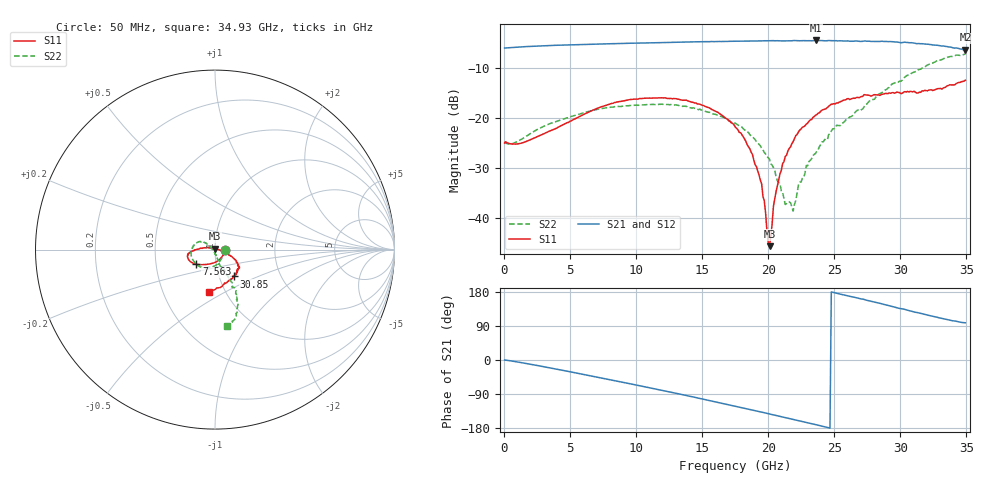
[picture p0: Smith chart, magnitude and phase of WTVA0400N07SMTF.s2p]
! 50 ohm 2-Port S-parameters measured by Modelithics Inc support@modelithics.com  Tampa, FL USA 813-866-6335 (February 2024)
! Smiths Interconnect,  4dB P/N: WTVA0400N07SMTF, Temperature: -25 C
! Board: 10 mil Rogers 4350B, Mounting Pad Dimensions: Length: 15 mils, Width: 25 mils, Gap: 40 mils.
# Hz S RI R 50
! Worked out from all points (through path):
!   352 points, 50 MHz to 34.93 GHz, reference 50 ohm
!   highest |S21| = -4.56 dB at 23.58 GHz (marker M1); lowest = -6.4 dB at 34.93 GHz (marker M2)
!   group delay of S21, straight-line fit = 21.3 ps
!   lowest |S11| = -45.6 dB at 20.1 GHz (marker M3), VSWR 1.01, Z = 50.1 + j0.521 ohm
!   |S11| at or under -10 dB: start of sweep to end of sweep
!   |S22| runs from -38.6 to -7.3 dB; largest |S21 - S12| = 0.0056
!   S11 on the Smith chart (normalised r, x): 50 MHz: 1.12, -0.01; 7.563 GHz: 0.80, -0.13; 30.85 GHz: 1.18, -0.36; 34.93 GHz: 0.84, -0.42
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5e7  0.0563 -0.00229  0.4972 -0.0006  0.4965 -0.000787  0.0576 -0.00224
5.8715e9  -0.0645 -0.0838  0.4309 -0.3249  0.4301 -0.3248  -0.0439 -0.1015
7.563e9  -0.1033 -0.081  0.3607 -0.411  0.3594 -0.4112  -0.0769 -0.0984
1.1742e10  -0.1525 -0.0435  0.1123 -0.5509  0.1107 -0.5505  -0.1305 -0.0407
1.5125e10  -0.132 -0.0104  -0.1366 -0.5585  -0.1379 -0.5575  -0.1143 0.0277
1.7513e10  -0.0805 0.0075  -0.3085 -0.4936  -0.3096 -0.4921  -0.0773 0.043
1.86075e10  -0.0481 0.0103  -0.3805 -0.4428  -0.3807 -0.4417  -0.0558 0.0391
1.9503e10  -0.0194 0.0105  -0.4318 -0.3953  -0.4322 -0.3938  -0.0401 0.0293
1.9702e10  -0.0121 0.00869  -0.4445 -0.3842  -0.4446 -0.383  -0.0374 0.0256
2.00005e10  -0.000736 0.00571  -0.4601 -0.3652  -0.4601 -0.364  -0.0337 0.0215
2.01e10  0.000821 0.0052  -0.4654 -0.3593  -0.4654 -0.3582  -0.0325 0.0212
2.03985e10  0.0129 0.00285  -0.4819 -0.339  -0.4823 -0.337  -0.0279 0.0155
2.0896e10  0.0275 -0.00345  -0.5029 -0.3028  -0.5031 -0.301  -0.0207 0.00691
2.1294e10  0.0402 -0.00911  -0.5161 -0.2762  -0.5165 -0.2741  -0.0137 -0.000515
2.1891e10  0.0561 -0.0151  -0.541 -0.2348  -0.541 -0.2329  -0.00695 -0.00949
2.2289e10  0.069 -0.0219  -0.5521 -0.2017  -0.5523 -0.1993  -0.00112 -0.0213
2.33835e10  0.0933 -0.0388  -0.5773 -0.1164  -0.5768 -0.1147  0.00875 -0.0411
2.35825e10  0.0972 -0.043  -0.583 -0.1  -0.5825 -0.0985  0.0107 -0.043
2.51745e10  0.1208 -0.0727  -0.5871 0.0385  -0.5862 0.0404  0.023 -0.0812
2.91545e10  0.1231 -0.1281  -0.4622 0.3448  -0.4598 0.3466  0.0905 -0.1796
3.0846e10  0.1057 -0.1493  -0.3517 0.4381  -0.349 0.4392  0.1206 -0.2511
3.49255e10  -0.0332 -0.2352  -0.0677 0.4748  -0.0632 0.4747  0.0679 -0.4281
